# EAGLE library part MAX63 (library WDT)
MAX6369-MAX6374 Maxim Watch Doc Timer datasheet
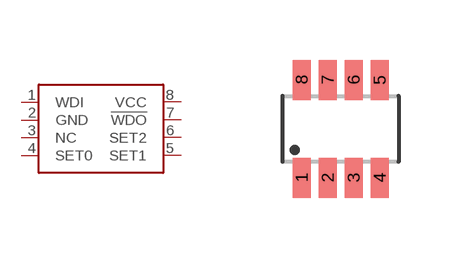
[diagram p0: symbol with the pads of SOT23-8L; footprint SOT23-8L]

Designator prefix U

## MAX6369  [SOT23-8L]
1  WDI
2  GND
3  NC
4  SET0
5  SET1
6  SET2
7  !WDO
8  VCC

## MAX6370  [SOT23-8L]
Pads as for SOT23-8L

## MAX6371  [SOT23-8L]
Pads as for SOT23-8L

## MAX6372  [SOT23-8L]
Pads as for SOT23-8L

## MAX6373  [SOT23-8L]
Pads as for SOT23-8L

## MAX6374  [SOT23-8L]
Pads as for SOT23-8L

## Footprint SOT23-8L (pad centres in mm)
SC70/SOT23-8 Source: http://datasheets.maxim-ic.com/en/ds/MAX4335-MAX4338.pdf
smd 0.45 x 1: 1 -0.975,-1.225; 2 -0.325,-1.225; 3 0.325,-1.225; 4 0.975,-1.225; 5 0.975,1.225; 6 0.325,1.225; 7 -0.325,1.225; 8 -0.975,1.225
